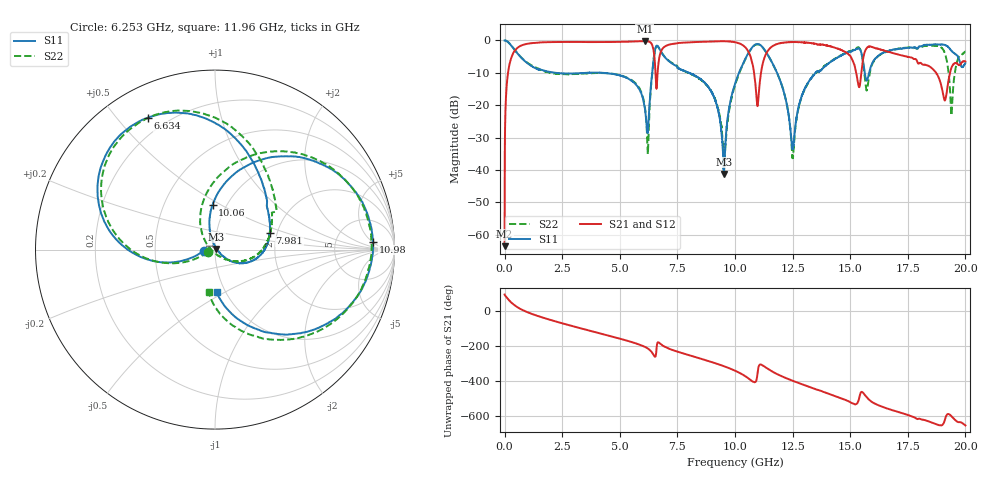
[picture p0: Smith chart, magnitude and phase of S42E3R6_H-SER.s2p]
! Created Wed Nov 25 21:44:03 2020
# khz S ma R 50
! 2 Port Network Data from SP1.SP block
! freq  magS11  angS11  magS21  angS21  magS12  angS12  magS22  angS22
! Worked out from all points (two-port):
!   20001 points, 300 kHz to 20 GHz, reference 50 ohm
!   highest |S21| = -0.20 dB at 6.082 GHz (marker M1); lowest = -63.5 dB at 300 kHz (marker M2)
!   |S21| within 3 dB of the highest: 435.1 MHz to 6.469 GHz (6.034 GHz wide, 175 % of centre); 6.799 GHz to 10.56 GHz (3.763 GHz wide, 43.3 % of centre)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
!   lowest |S11| = -41.2 dB at 9.519 GHz (marker M3), VSWR 1.02, Z = 50.8 + j0.399 ohm
!   |S11| at or under -10 dB: 4.282 GHz to 6.401 GHz (2.118 GHz wide, 39.7 % of centre); 8.009 GHz to 10.17 GHz (2.163 GHz wide, 23.8 % of centre); 11.82 GHz to 13.49 GHz (1.667 GHz wide, 13.2 % of centre)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
!   |S22| runs from -36.6 to 0.0 dB; largest |S21 - S12| = 0.02
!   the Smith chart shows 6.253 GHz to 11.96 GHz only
!   S11 on the Smith chart (normalised r, x): 6.253 GHz: 0.88, -0.01; 6.634 GHz: 0.13, +0.60; 7.981 GHz: 1.83, +0.38; 10.06 GHz: 0.86, +0.46; 10.98 GHz: 14, +5; 11.96 GHz: 0.91, -0.46
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300  0.9996 -0.2  0.0006688 91.3  0.0007504 94.8  0.9999 -0.2
121300  0.9628 -19.8  0.2644 69.9  0.2651 69.9  0.9629 -19.8
397300  0.7454 -56.4  0.6599 34.1  0.661 34.1  0.7475 -56.1
1306300  0.3784 -115.7  0.9178 -24.8  0.9168 -24.8  0.3887 -114.8
3334300  0.3134 164.1  0.9467 -102.3  0.9465 -102.3  0.3074 170.4
6082300  0.09259 79.7  0.9767 153.4  0.9753 153.4  0.09706 66.6
6253300  0.06203 -174.6  0.9619 140.2  0.9618 140.3  0.04245 -163.8
6634300  0.825 117.0  0.2919 176.2  0.2917 175.8  0.821 113.8
6667300  0.8 107.7  0.4116 179.2  0.4115 178.9  0.7982 104.0
7981300  0.319 16.8  0.9349 106.4  0.9321 106.7  0.3159 15.4
9519300  0.008715 26.8  0.9717 42.6  0.9753 42.6  0.01633 -110.9
1.00003e7  0.2144 96.4  0.9394 17.2  0.9384 17.1  0.2043 113.6
1.00623e7  0.2484 93.2  0.9298 13.4  0.9271 13.4  0.2391 108.8
1.09783e7  0.8815 2.9  0.0971 3.7  0.0973 4.4  0.8725 2.4
1.19623e7  0.2381 -87.6  0.9071 -10.6  0.909 -10.7  0.2408 -98.5
1.25083e7  0.02169 -24.3  0.9442 -40.4  0.9451 -40.7  0.01562 -38.3
1.33343e7  0.2685 13.3  0.9051 -80.6  0.9077 -80.4  0.2691 0.5
1.53713e7  0.7561 -106.6  0.1966 -148.9  0.1953 -149.7  0.7791 -110.5
1.66673e7  0.6894 -109.5  0.6685 159.1  0.6528 159.1  0.6886 -113.1
1.84553e7  0.8547 -179.2  0.3944 85.6  0.3943 86.1  0.834 174.5
1.94013e7  0.6865 125.2  0.3832 116.6  0.3824 116.6  0.07198 157.1
2e7  0.4469 129.2  0.4754 65.2  0.4778 66.0  0.6717 154.1
